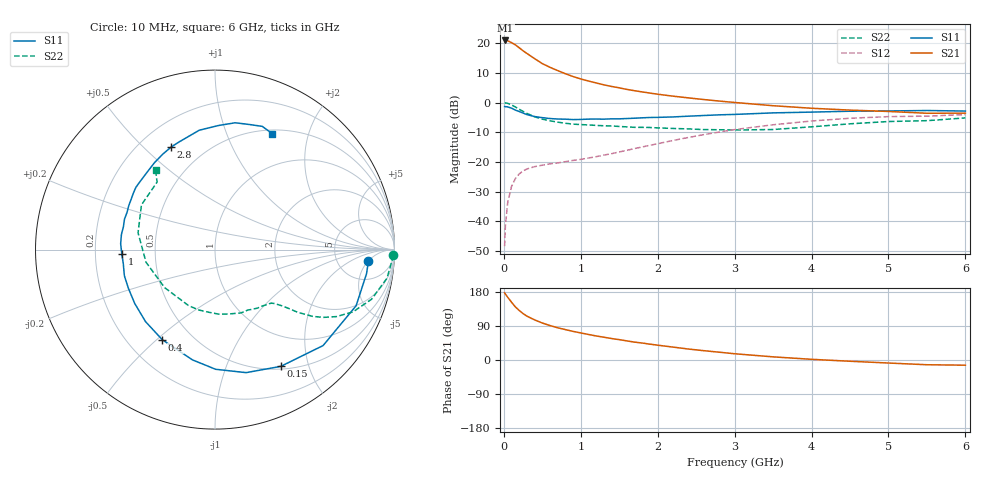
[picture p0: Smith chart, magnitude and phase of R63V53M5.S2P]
! SIEMENS Small Signal Semiconductors
! BFR193
! Si NPN RF Bipolar Junction Transistor in SOT23
! VCE = 3.5 V  IC = 3.5 mA
! Common Emitter S-Parameters:  May  1996
# GHz  S  MA  R  50
!  f  S11  S21  S12  S22
! GHz  MAG  ANG  MAG  ANG  MAG  ANG  MAG  ANG
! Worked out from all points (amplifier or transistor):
!   36 points, 10 MHz to 6 GHz, reference 50 ohm
!   highest |S21| = 20.9 dB at 20 MHz (marker M1)
!   |S21| within 3 dB of that: start of sweep to 226.1 MHz
!   unconditionally stable (mu >= 1): 982.9 MHz to 2.031 GHz
!   at 250 MHz: K = 0.33, MSG = 20.2 dB, |S12| = -23.0 dB
!   at 1.4 GHz: K = 1.08, MAG = 9.6 dB, |S12| = -17.2 dB
!   at 6 GHz: K = 0.98, MSG = 0.2 dB, |S12| = -4.0 dB
!   S11 on the Smith chart (normalised r, x): 10 MHz: 11, -5; 150 MHz: 0.54, -1.58; 400 MHz: 0.34, -0.52; 1 GHz: 0.32, -0.02; 2.8 GHz: 0.33, +0.61; 6 GHz: 0.55, +1.47
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0.01  0.8573 -4.3  11.02 177.4  0.0038 91.5  0.9944 -1.8
0.02  0.855 -9.0  11.15 174.0  0.0082 85.4  0.9872 -3.8
0.05  0.8461 -21.7  11.03 165.6  0.0206 77.8  0.9718 -9.4
0.1  0.8053 -41.6  10.24 152.5  0.0386 68.4  0.9151 -17.6
0.15  0.7467 -60.6  9.409 140.0  0.0525 60.4  0.8434 -24.3
0.2  0.7071 -75.8  8.4 130.7  0.0627 54.6  0.7724 -28.9
0.25  0.6668 -89.7  7.462 122.5  0.0705 49.8  0.7109 -32.1
0.3  0.6273 -101.5  6.733 115.7  0.0761 46.9  0.658 -34.4
0.4  0.5818 -120.3  5.508 105.9  0.0832 43.3  0.5772 -37.2
0.5  0.5574 -134.0  4.542 97.6  0.0881 41.7  0.5259 -38.6
0.6  0.5386 -146.2  3.934 90.9  0.0928 41.7  0.4941 -39.7
0.7  0.5284 -156.0  3.465 85.1  0.0962 42.8  0.4682 -41.0
0.8  0.5255 -163.9  3.066 80.2  0.101 44.3  0.4484 -42.1
1  0.5198 -177.5  2.504 71.4  0.1103 48.2  0.4263 -45.1
1.1  0.5267 176.4  2.309 67.4  0.1164 49.9  0.4198 -47.2
1.6  0.5392 153.0  1.667 50.4  0.1568 57.7  0.3894 -59.0
2.2  0.5731 131.5  1.284 34.0  0.2299 59.1  0.3665 -78.4
2.8  0.6217 113.1  1.061 20.6  0.3188 54.1  0.3484 -104.9
3.5  0.6709 97.5  0.886 8.3  0.4229 42.8  0.3517 -143.0
4.5  0.7154 81.0  0.747 -3.3  0.5445 24.6  0.4388 167.7
5.5  0.7354 69.0  0.661 -12.5  0.5912 6.5  0.4957 130.6
6  0.7201 63.6  0.664 -13.7  0.6276 1.5  0.5517 126.9
